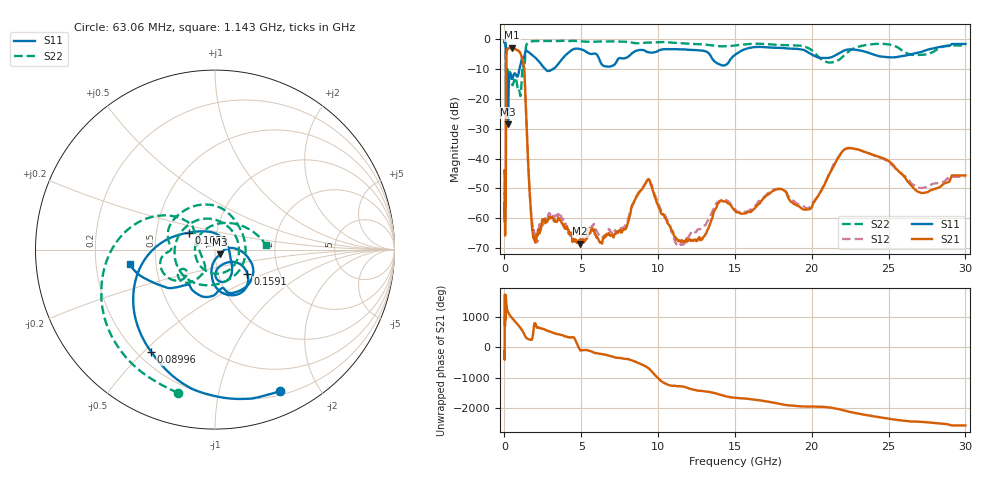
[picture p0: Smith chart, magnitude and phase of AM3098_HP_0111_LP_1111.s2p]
! Date/Time: Thu, Feb 28, 2019 8:39 AM
! Network Analyzer: Agilent Technologies E8364B Rev: A.07.50.67
! Sweep from 0.010 to 30.000 GHz, 1601 Points, Sweep Type: LOG
! Power Supply: 5.022 V, 0.002 A
# Hz S DB R 50
!freq MagS11 AngS11 MagS21 AngS21 MagS12 AngS12 MagS22 AngS22
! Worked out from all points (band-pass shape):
!   1601 points, 10 MHz to 30 GHz, reference 50 ohm
!   highest |S21| = -2.76 dB at 498 MHz (marker M1); lowest = -68.6 dB at 4.927 GHz (marker M2)
!   |S21| within 3 dB of the highest: 122.7 MHz to 1.113 GHz (990.5 MHz wide, 160 % of centre)
!   lowest |S11| = -28.5 dB at 237.5 MHz (marker M3), VSWR 1.08, Z = 52.7 - j2.73 ohm
!   |S11| at or under -10 dB: 102.2 MHz to 973.1 MHz (871 MHz wide, 162 % of centre); 2.666 GHz to 3.156 GHz (490.1 MHz wide, 16.8 % of centre)
!   |S22| runs from -21.6 to -0.5 dB; largest |S21 - S12| = 0.01
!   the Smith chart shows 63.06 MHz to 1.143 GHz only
!   S11 on the Smith chart (normalised r, x): 63.06 MHz: 0.24, -1.53; 89.96 MHz: 0.25, -0.53; 105.1 MHz: 0.73, +0.14; 159.1 MHz: 1.38, -0.39; 1.143 GHz: 0.35, -0.07
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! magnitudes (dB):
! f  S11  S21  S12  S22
! 10 MHz  -0.3  -43.9  -45.3  -0.6
! 38.04 MHz  -0.4  -60.3  -58.4  -1.0
! 63.06 MHz  -1.2  -53.6  -52.5  -1.7
! 89.96 MHz  -3.5  -46.3  -46.8  -3.8
! 105.1 MHz  -15.2  -14.9  -15.0  -19.2
! 144.7 MHz  -19.6  -4.0  -4.0  -14.1
! 159.1 MHz  -13.0  -3.7  -3.7  -11.9
! 237.5 MHz  -28.5  -3.0  -3.0  -11.9
! 311.2 MHz  -12.6  -2.9  -2.8  -11.3
! 498 MHz  -13.2  -2.8  -2.7  -15.0
! 550.5 MHz  -12.7  -2.9  -2.9  -15.2
! 1.143 GHz  -6.3  -6.3  -6.3  -10.9
! 1.308 GHz  -5.4  -12.2  -12.1  -8.9
! 1.802 GHz  -5.2  -63.2  -61.0  -0.6
! 2.084 GHz  -6.5  -66.7  -68.0  -0.5
! 4.927 GHz  -3.3  -68.6  -66.5  -0.6
! 7.926 GHz  -6.2  -63.3  -61.7  -0.8
! 9.302 GHz  -4.3  -47.3  -47.0  -1.1
! 12.56 GHz  -3.6  -67.6  -63.9  -1.6
! 19.7 GHz  -4.2  -57.1  -56.7  -2.7
! 22.78 GHz  -3.4  -36.7  -36.7  -2.9
! 30 GHz  -1.5  -45.7  -46.1  -2.0
